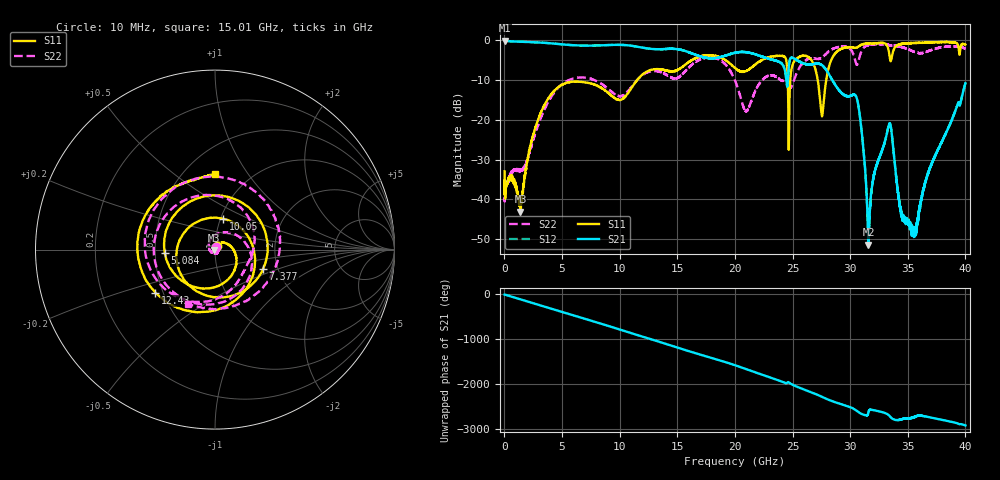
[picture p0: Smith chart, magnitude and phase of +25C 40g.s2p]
!Keysight Technologies,N5234A,MY52241180,A.10.60.03
!Date: Tuesday, February 27, 2024 08:40:13
!Correction: S11(Full 2 Port(1,2))
!S21(Full 2 Port(1,2))
!S12(Full 2 Port(1,2))
!S22(Full 2 Port(1,2))
!S2P File: Measurements: S11, S21, S12, S22:
# Hz S  dB  R 50
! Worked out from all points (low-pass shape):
!   6401 points, 10 MHz to 40 GHz, reference 50 ohm
!   highest |S21| = -0.06 dB at 16.25 MHz (marker M1); lowest = -51.4 dB at 31.58 GHz (marker M2)
!   |S21| within 3 dB of the highest: start of sweep to 16.04 GHz; 20.17 GHz to 21.12 GHz (945.4 MHz wide, 4.58 % of centre)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
!   lowest |S11| = -43.1 dB at 1.385 GHz (marker M3), VSWR 1.01, Z = 49.3 - j0.188 ohm
!   |S11| at or under -10 dB: start of sweep to 11.51 GHz; 24.58 GHz to 24.8 GHz (218.6 MHz wide, 0.885 % of centre); 27.19 GHz to 27.92 GHz (732.2 MHz wide, 2.66 % of centre)
!   |S22| runs from -40.6 to -0.9 dB; largest |S21 - S12| = 0.0074
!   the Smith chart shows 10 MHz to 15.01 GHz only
!   S11 on the Smith chart (normalised r, x): 10 MHz: 1.02, +0.04; 5.084 GHz: 0.56, -0.02; 7.377 GHz: 1.67, -0.40; 10.05 GHz: 1.03, +0.37; 12.43 GHz: 0.45, -0.26; 15.01 GHz: 0.70, +0.72
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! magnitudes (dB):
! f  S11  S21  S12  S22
! 10 MHz  -33.0  -0.1  0.0  -36.4
! 16.25 MHz  -38.9  -0.1  -0.1  -40.6
! 1.385 GHz  -43.1  -0.4  -0.4  -32.7
! 2.884 GHz  -20.1  -0.5  -0.5  -21.5
! 5.084 GHz  -11.1  -1.0  -1.0  -10.8
! 6.677 GHz  -10.5  -1.3  -1.3  -9.4
! 7.377 GHz  -10.8  -1.3  -1.3  -9.6
! 10.05 GHz  -15.0  -1.2  -1.2  -14.1
! 12.43 GHz  -7.8  -2.1  -2.1  -8.0
! 13.34 GHz  -7.3  -2.2  -2.2  -7.8
! 15.01 GHz  -7.5  -2.2  -2.2  -9.5
! 20 GHz  -7.0  -3.1  -3.1  -10.2
! 21 GHz  -7.7  -3.0  -3.0  -17.8
! 26.67 GHz  -5.1  -6.0  -6.0  -4.6
! 27.57 GHz  -19.1  -6.3  -6.3  -4.3
! 28.51 GHz  -4.1  -10.3  -10.3  -2.1
! 30.53 GHz  -1.9  -14.2  -14.2  -5.9
! 31.58 GHz  -0.8  -51.4  -51.1  -1.2
! 33.34 GHz  -2.5  -21.6  -21.5  -1.2
! 34.43 GHz  -1.0  -43.0  -43.0  -1.7
! 35.54 GHz  -0.7  -49.1  -47.8  -2.9
! 40 GHz  -1.0  -10.8  -10.8  -2.1
